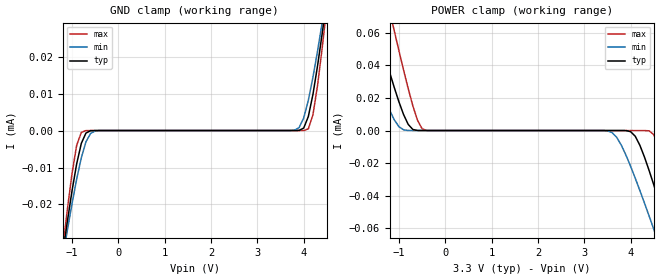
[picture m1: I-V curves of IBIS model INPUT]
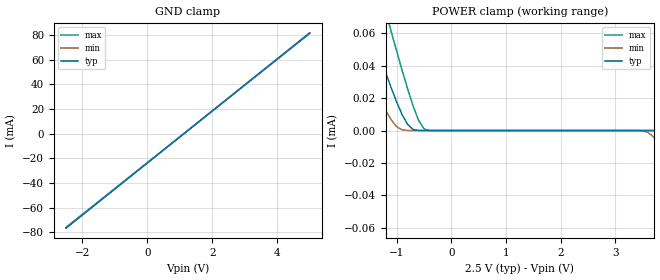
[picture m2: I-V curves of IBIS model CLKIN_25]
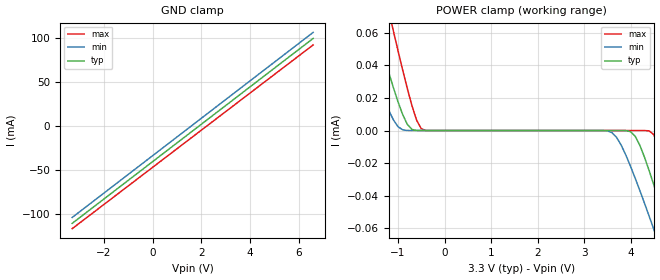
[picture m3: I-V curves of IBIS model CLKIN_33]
|   DIODES INCORPORATED
|   IBIS Model of PI6C5922504
|   Product Family: 6C
|   TQFN-16 Package (ZH)
[IBIS Ver] 3.2
[Comment char] |_char
[File Name] pi6c5922504_zh_revb.ibs
[File Rev] 1.1
[Source] File originated at Diodes Incorporated.
[Date] 09/19/2019
[Disclaimer] (C) Copyright DIODES INCORPORATED
   All rights reserved
  Diodes Incorporated hereby grants the user of
  this IBIS model a non-exclusive, nontransferable license to
  use this IBIS model under the following terms.
  This IBIS model is provided on an "AS IS" basis and Diodes
  makes absolutely no warranty with respect to the information
  contained herein. DIODES DISCLAIMS AND CUSTOMER WAIVES ALL
  WARRANTIES, EXPRESSED OR IMPLIED, INCLUDING WARRANTIES OF
  MERCHANTABILITY OR FITNESS FOR A PARTICULAR PURPOSE. The
  entire risk as to quality and performance is with the customer.
  Accordingly, in no event shall the company be liable for any
  damages, whether in contract or tort, including any lost
  profits or other incidental, consequential, exemplary, or
  punitive damages arising out of the use or application of the
  IBIS model provided in this package. Further, Diodes reserves
  the right to make changes without notice to any product herein
  to improve reliability, function, or design. Diodes does not
  convey any license under patent rights or any other intellectual
  property rights, including those of third parties.
  The user is granted this license only to use the IBIS model
  and is not granted rights to sell, load, rent, lease or license
  the IBIS model in whole or in part, or in modified form to anyone
  other than user. User may modify the IBIS model to suit its specific
  application but rights to derivative works and such modifications
  shall belong to Diodes.
  Diodes is not obligated to provide maintenance or support
  for the licensed IBIS model.
  Contact Diodes at ATTN: APPLICATION ENGINEERING / IBIS MODELS
  1545 Barber Ln. Milpitas, CA 95035
[Component] PI6C5922504
[Manufacturer] Diodes Incorporated.
[Package]
| variable   typ   min  max
R_pkg   0.03869ohm   NA   NA
L_pkg   2.64482nH   NA   NA
C_pkg   0.19279pF   NA   NA
[Pin]   signal_name   model_name   R_pin   L_pin   C_pin
1   Q1+   OUTPUT   0.05182  3.00059n  0.31036p
2   Q1-   OUTPUT   0.04933  2.81497n  0.25618p
3   Q2+   OUTPUT   0.04933  2.81497n  0.25618p
4   Q2-   OUTPUT   0.05182  3.00059n  0.31036p
5   Q3+   OUTPUT   0.05182  3.00059n  0.31036p
6   Q3-   OUTPUT   0.04933  2.81497n  0.25618p
7   VDD   POWER   0.04933  2.81497n  0.25618p
8   EN   INPUT   0.05182  3.00059n  0.31036p
9   REF_IN-   CLKIN   0.05182  3.00059n  0.31036p
10   VREF-AC   NC   0.04933  2.81497n  0.25618p
11   VTH   NC   0.04933  2.81497n  0.25618p
12   REF_IN+   CLKIN   0.05182  3.00059n  0.31036p
13   GND   GND   0.05182  3.00059n  0.31036p
14   VDD   POWER   0.04933  2.81497n  0.25618p
15   Q0+   OUTPUT   0.04933  2.81497n  0.25618p
16   Q0-   OUTPUT   0.05182  3.00059n  0.31036p
[Diff Pin]  inv_pin vdiff   tdelay_typ tdelay_min tdelay_max
2   1   NA   0ns   0ns   0ns
4   3   NA   0ns   0ns   0ns
6   5   NA   0ns   0ns   0ns
16   15   NA   0ns   0ns   0ns
| Model DIFFOUT
[Model Selector]   OUTPUT
LVDS_33   3.3 volt VDD
LVDS_25   2.5 volt VDD
| Model CLKIN
[Model Selector]   CLKIN
CLKIN_33   3.3 volt VDD
CLKIN_25   2.5 volt VDD
| Models and submodels in the file (5): INPUT (Input), CLKIN_25 (Input), CLKIN_33 (Input), LVDS_25 (Output), LVDS_33 (Output)
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|   Model INPUT
[Model] INPUT
Model_type Input
Vinl = 800mV
Vinh = 2.00V
| variable   typ   min   max
C_comp   0.436pF   0.433pF   0.438pF
[Voltage Range]   3.300V   3.135V   3.465V
[GND Clamp Reference]   0.000V   0.000V   0.000V
[POWER Clamp Reference]   3.300V   3.135V   3.465V
[temperature range]   25   85   -40
[GND Clamp]
| Voltage   I(typ)   I(min)   I(max)
-3.3V     -239.4uA   -209.3uA   -287.2uA
-1.2V     -33.2uA    -34.4uA    -31.89uA
-1.1V     -24.47uA   -26.92uA   -21.23uA
-900mV    -9.002uA   -13.13uA   -4.02uA
-700mV    -691.5nA   -3.066uA   -12.48nA
-400mV    -38.89pA   -6.45nA    -8.204pA
3.8V      984.7pA    78.9nA     9.147pA
4.1V      3.785uA    8.176uA    450.5nA
4.2V      9.811uA    14.44uA    4.276uA
4.4V      26.33uA    29.28uA    22.46uA
4.5V      35.61uA    37.31uA    33.62uA
6.6V      255uA      225.3uA    301.3uA
[POWER Clamp]   |Note: Vtable = Vcc - Voutput
| Voltage   I(typ)   I(min)   I(max)
-3.3V     255uA      194.9uA    344.5uA
-1.9V     106.2uA    68.71uA    162.2uA
-1.5V     65.12uA    34.88uA    111uA
-1.2V     35.61uA    12.45uA    73.34uA
-800mV    3.785uA    34.46nA    25.73uA
-400mV    31.28pA    7.027pA    29.8nA
3.6V      -8.401pA   -1.257uA   -6.48pA
4.1V      -3.477uA   -29.13uA   -8.625pA
4.4V      -24.47uA   -52.38uA   -202.4nA
4.8V      -60.97uA   -84.96uA   -28.62uA
5.1V      -89.87uA   -110uA     -62.74uA
6.6V      -239.4uA   -237.7uA   -246.1uA
|   Model CLKIN_25
[Model] CLKIN_25
Model_type Input
Vinl = 1.10V
Vinh = 1.30V
| variable   typ   min   max
C_comp   0.436pF   0.433pF   0.438pF
[Voltage Range]   2.500V   2.375V   2.625V
[GND Clamp Reference]   0.000V   0.000V   0.000V
[POWER Clamp Reference]   2.500V   2.375V   2.625V
[temperature range]   25   85   -40
[GND Clamp]
| Voltage   I(typ)   I(min)   I(max)
-2.5V     -76.62mA   -76.74mA   -76.12mA
4V        60.61mA    60.61mA    60.24mA
4.7V      75.38mA    75.39mA    74.92mA
5V        81.71mA    81.72mA    81.21mA
[POWER Clamp]   |Note: Vtable = Vcc - Voutput
| Voltage   I(typ)   I(min)   I(max)
-2.5V     169.5uA    122uA      240uA
-1.9V     106.2uA    68.71uA    162.2uA
-1.5V     65.12uA    34.88uA    111uA
-1.1V     26.33uA    6.551uA    61.02uA
-700mV    663.5nA    1.759nA    15.2uA
-400mV    31.28pA    7.027pA    29.8nA
3.5V      -7.412pA   -204.5nA   -6.08pA
3.7V      -38.89pA   -4.16uA    -6.88pA
4V        -691.5nA   -21.87uA   -8.081pA
4.5V      -33.2uA    -60.41uA   -2.486uA
4.8V      -60.97uA   -84.96uA   -28.62uA
5V        -80.16uA   -101.6uA   -51.09uA
|   Model CLKIN_33
[Model] CLKIN_33
Model_type Input
Vinl = 1.30V
Vinh = 2.50V
| variable   typ   min   max
C_comp   0.436pF   0.433pF   0.438pF
[Voltage Range]   3.300V   2.970V   3.630V
[GND Clamp Reference]   0.000V   0.000V   0.000V
[POWER Clamp Reference]   3.300V   2.970V   3.630V
[temperature range]   25   85   -40
[GND Clamp]
| Voltage   I(typ)   I(min)   I(max)
-3.3V     -110.2mA   -103.5mA   -116.2mA
-3.2V     -108.1mA   -101.4mA   -114.1mA
-3V       -103.8mA   -97.15mA   -109.9mA
6.6V      99.29mA    106.1mA    91.94mA
[POWER Clamp]   |Note: Vtable = Vcc - Voutput
| Voltage   I(typ)   I(min)   I(max)
-3.3V     255uA      194.9uA    344.5uA
-1.9V     106.2uA    68.71uA    162.2uA
-1.5V     65.12uA    34.88uA    111uA
-1.2V     35.61uA    12.45uA    73.34uA
-800mV    3.785uA    34.46nA    25.73uA
-400mV    31.28pA    7.027pA    29.8nA
3.6V      -8.401pA   -1.257uA   -6.48pA
4.1V      -3.477uA   -29.13uA   -8.625pA
4.4V      -24.47uA   -52.38uA   -202.4nA
4.8V      -60.97uA   -84.96uA   -28.62uA
5.1V      -89.87uA   -110uA     -62.74uA
6.6V      -239.4uA   -237.7uA   -246.1uA
